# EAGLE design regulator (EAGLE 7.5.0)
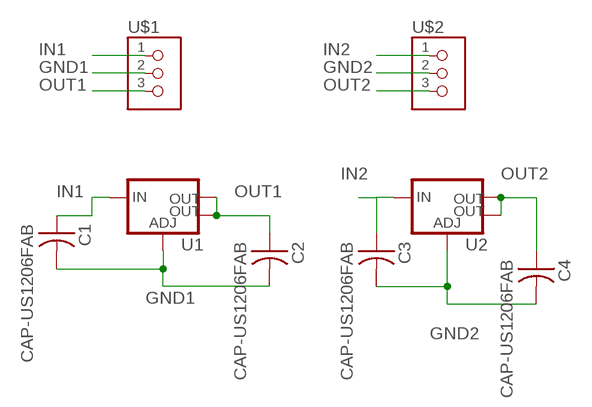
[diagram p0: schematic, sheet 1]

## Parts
C1  CAP-US1206FAB  [C1206FAB]
C2  CAP-US1206FAB  [C1206FAB]
C3  CAP-US1206FAB  [C1206FAB]
C4  CAP-US1206FAB  [C1206FAB]
U1  V_REG_LM1117SOT223  [SOT223]
U2  V_REG_LM1117SOT223  [SOT223]
U$1  TERM-1X03'-FABLAB'  [ED555DS-3DS]
U$2  TERM-1X03'-FABLAB'  [ED555DS-3DS]

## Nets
GND1: C1.2 C2.2 U1.1(ADJ) U$1.2
GND2: C3.2 C4.2 U2.1(ADJ) U$2.2
IN1: C1.1 U1.3(IN) U$1.1
IN2: C3.1 U2.3(IN) U$2.1
OUT1: C2.1 U1.2(OUT) U1.4(OUT) U$1.3
OUT2: C4.1 U2.2(OUT) U2.4(OUT) U$2.3

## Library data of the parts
C1-C4 = fab:CAP-US
U1 U2 = fab:V_REG_LM1117: Voltage Regulator LM1117 Standard adjustable voltage regulator but in SMD form. Spark Fun Electronics SKU : COM-00595; PROD_ID: VREG-08170
U$1 U$2 = fab:TERM-1X03: 3.5mm terminal block, 3 positions ED555-3DS as found in the fablab inventory. Made by Zaerc.

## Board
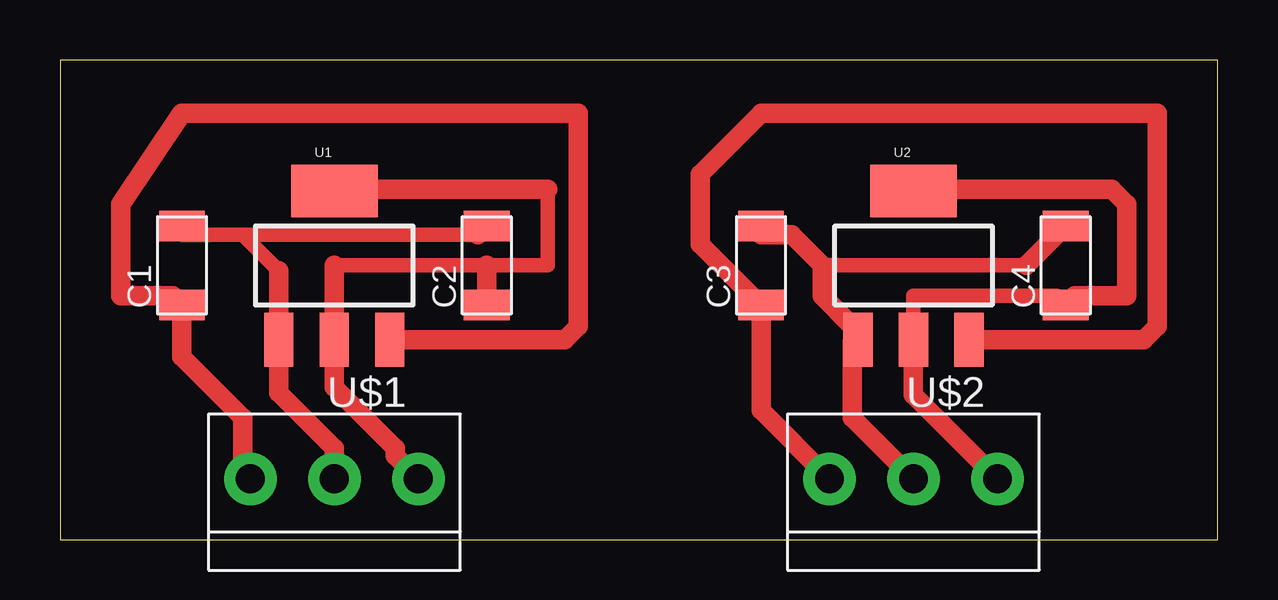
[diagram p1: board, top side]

Size 48.24 x 19.99 mm. Coordinates in mm from the lower left corner, seen from the top.
Outline: 0,0 48.24,0 48.24,19.99 0,19.99 0,0
Copper layers (1*16): Top 0.035mm / dielectric 1.5mm / Bottom 0.035mm
Design rules "default *": minimum track width 10mil, minimum drill 24mil, track to track 16mil, track to pad 16mil, pad to pad 16mil, via to via 16mil, smd to smd 16mil, copper to edge 40mil, drill to drill 8mil, minimum pad ring 10mil, minimum via ring 8mil, stop-mask expansion 4mil, vias tented up to drill 0mil, thermal gap 10mil

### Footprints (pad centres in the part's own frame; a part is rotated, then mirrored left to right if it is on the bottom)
C1206FAB = smd 1.27 x 1.905: 1 -1.651,0; 2 1.651,0
SOT223 = smd 1.219 x 2.235: 1 -2.311,-3.099; 2 0,-3.099; 3 2.311,-3.099 | smd 3.6 x 2.2: 4 0,3.099
ED555DS-3DS = drill 1.2 pad 2.184: 1 -3.5,0; 2 0,0; 3 3.5,0

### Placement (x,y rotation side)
C1  5.08,11.43 90 top
C2  17.78,11.43 90 top
C3  29.21,11.43 90 top
C4  41.91,11.43 90 top
U1  11.43,11.43 0 top
U2  35.56,11.43 0 top
U$1  11.43,2.54 0 top
U$2  35.56,2.54 0 top

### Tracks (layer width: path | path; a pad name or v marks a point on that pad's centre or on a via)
GND1
  Top 0.254: 5.08,12.7 C1.2 | 8.89,8.89 U1.1 8.89,8.25 | 17.78,12.7 C2.2
  Top 0.61: 7.62,12.7 17.4,12.7 | 5.08,12.7 7.62,12.7 | 7.62,12.7 9.12,11.2
  Top 0.813: 17.4,12.7 C2.2 | 9.12,11.2 U1.1 9.12,6.12 11.43,3.81 U$1.2
GND2
  Top 0.254: 29.21,12.7 C3.2 | 33.02,8.89 U2.1 33.02,8.25 | 41.91,12.7 C4.2
  Top 0.61: 31.75,11.43 40.26,11.43
  Top 0.813: 29.21,12.7 30.48,12.7 31.75,11.43 31.75,10.16 33.02,8.89 | 40.26,11.43 C4.2 | 33.02,8.25 33.02,5.08 U$2.2
IN1
  Top 0.254: 13.97,8.25 U1.3
  Top 0.813: U$1.1 7.62,2.85 7.62,5.08 5.08,7.62 C1.1 4.7,10.16 2.54,10.16 2.54,13.97 5.08,17.78 21.59,17.78 21.59,8.89 21.03,8.33 U1.3
IN2
  Top 0.254: 38.1,8.25 U2.3
  Top 0.813: U$2.1 29.21,5.39 C3.1 26.67,12.32 26.67,15.24 29.21,17.78 45.72,17.78 45.72,8.89 45.16,8.33 U2.3
OUT1
  Top 0.254: 11.43,8.89 U1.2 11.43,7.62 | 11.43,14.6 U1.4 | 14.61,2.54 U$1.3
  Top 0.61: 11.43,11.43 17.78,11.43 20.32,11.43 20.32,14.6
  Top 0.813: 11.43,14.6 20.32,14.6 | 17.78,11.43 C2.1 | 11.43,11.43 11.43,7.62 11.43,6.35 13.97,3.81 13.97,3.5 U$1.3
OUT2
  Top 0.254: 35.56,8.89 U2.2 | 35.56,14.6 U2.4 | 41.91,10.16 C4.1
  Top 0.61: 35.56,8.89 35.56,10.16 41.53,10.16 C4.1
  Top 0.813: 35.56,14.6 43.81,14.6 44.45,13.97 44.45,10.16 42.29,10.16 C4.1 | U2.2 35.56,6.04 U$2.3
